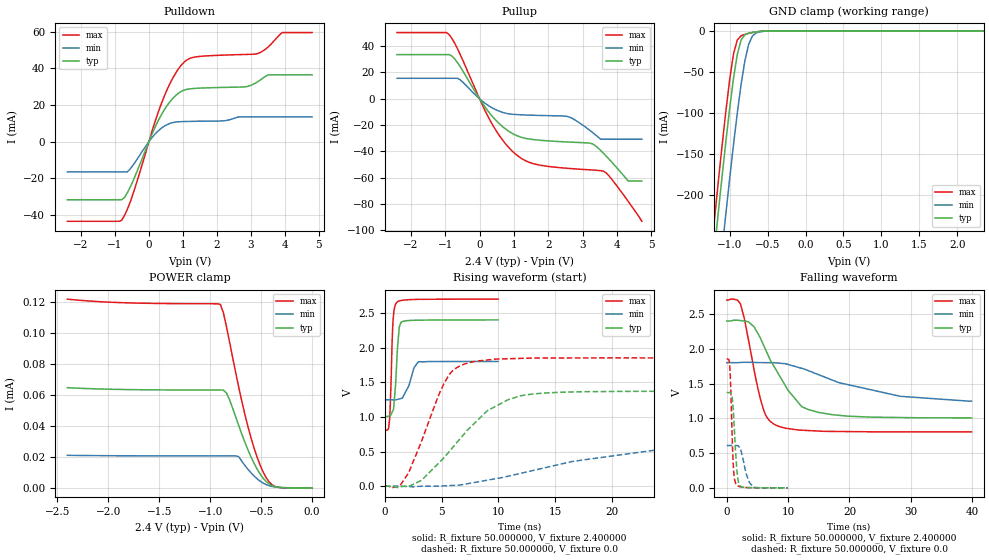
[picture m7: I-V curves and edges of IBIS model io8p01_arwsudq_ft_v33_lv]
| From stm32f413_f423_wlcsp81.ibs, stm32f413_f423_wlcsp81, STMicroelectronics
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|   Model io8p01_arwsudq_ft_v33_lv
[Model]  io8p01_arwsudq_ft_v33_lv
Model_type I/O
Polarity   Non-Inverting
Enable   Active-Low
Vinl =   0.720000V
Vinh =   1.680000V
Vmeas =  1.200000V
Cref =   50.000000pF
Rref =   100.000000M
Vref =   0.0V
C_comp   2.828400pF   2.771400pF   2.910300pF
[Temperature Range]   25.000000   0.125000k   -40.000000
[Pullup Reference]   2.400000V   1.800000V   2.700000V
[Pulldown Reference]   0.0V   0.0V   0.0V
[POWER Clamp Reference]   2.400000V   1.800000V   2.700000V
[GND Clamp Reference]   0.0V   0.0V   0.0V
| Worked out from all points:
|   slope of the pulldown table from 0 to 0.36 V, typ, clamps not added: 25 ohm
|   slope of the pullup table from 0 to 0.36 V, typ, clamps not added: 27.7 ohm
|   GND clamp passes 1 mA (typ) near -0.62 V on its own axis
|   rising waveform, R_fixture 50.000000, V_fixture 2.400000: 20-80 % time 323ps typ, 711ps min, 222ps max; typ from 1.01 V to 2.4 V
|   rising waveform, R_fixture 50.000000, V_fixture 0.0: 20-80 % time 4.72ns typ, 12.1ns min, 2.67ns max; typ from 0 V to 1.37 V
|   falling waveform, R_fixture 50.000000, V_fixture 2.400000: 20-80 % time 5.45ns typ, 13ns min, 2.68ns max; typ from 2.4 V to 1.01 V
|   falling waveform, R_fixture 50.000000, V_fixture 0.0: 20-80 % time 553ps typ, 1.05ns min, 408ps max; typ from 1.37 V to 0 V
[Pulldown]
|Voltage   I(typ)   I(min)   I(max)
-2.4V     -31.66mA   -16.51mA   -43.43mA
-800mV    -31.66mA   -16.51mA   -42.86mA
-480mV    -21.98mA   -13.17mA   -29.21mA
80mV      3.63mA     1.966mA    5.014mA
480mV     18.16mA    8.738mA    26.02mA
800mV     25.38mA    10.72mA    37.77mA
1.12V     28.53mA    11.02mA    44.6mA
2.8V      29.84mA    13.48mA    47.53mA
3.2V      32.65mA    13.48mA    48.04mA
3.52V     36.42mA    13.48mA    51.83mA
3.92V     36.42mA    13.48mA    59.49mA
4.8V      36.42mA    13.48mA    59.49mA
[Pullup]
|Voltage   I(typ)   I(min)   I(max)
-2.4V     33.57mA    15.57mA    50.34mA
-960mV    33.57mA    15.57mA    50.34mA
-800mV    32.45mA    15.57mA    45.78mA
-560mV    24.29mA    14.31mA    33.54mA
320mV     -11.75mA   -6.207mA   -17.08mA
960mV     -26.47mA   -11.82mA   -40.02mA
1.52V     -30.88mA   -12.51mA   -49.05mA
2.56V     -32.88mA   -13.49mA   -52.9mA
3.28V     -34.2mA    -25.51mA   -54.18mA
3.6V      -41.34mA   -30.76mA   -55mA
4.32V     -62.5mA    -30.76mA   -77.89mA
4.72V     -62.5mA    -30.76mA   -93.2mA
[GND_clamp]
|Voltage   I(typ)   I(min)   I(max)
-2.4V     -1.428A    -1.51A     -1.401A
-1.2V     -266.4mA   -356.3mA   -229.4mA
-1.15V    -221.3mA   -311mA     -184.1mA
-1.1V     -177.3mA   -266.4mA   -140mA
-1.05V    -134.8mA   -222.7mA   -97.97mA
-950mV    -58.22mA   -139.2mA   -28.55mA
-900mV    -29.03mA   -100.6mA   -11.27mA
-850mV    -11.41mA   -65.77mA   -6.067mA
-750mV    -2.852mA   -16.63mA   -3.179mA
-700mV    -1.914mA   -6.318mA   -2.181mA
-600mV    -750uA     -1.167mA   -738.3uA
2.35V     0A         0A         0A
[POWER_clamp]
|Voltage   I(typ)   I(min)   I(max)
-2.4V     64.71uA    21.03uA    121.9uA
-1.86V    63.55uA    20.74uA    119.6uA
-900mV    63.18uA    20.63uA    118.5uA
-870mV    63.14uA    20.63uA    113.2uA
-840mV    61.36uA    20.62uA    104.3uA
-720mV    40.37uA    20.18uA    65.28uA
-630mV    24.69uA    12.08uA    39.85uA
-540mV    12.26uA    5.907uA    20uA
-480mV    6.236uA    3.061uA    10.23uA
-420mV    2.4uA      1.365uA    3.726uA
-360mV    667.9nA    564nA      839.6nA
0V        0A         0A         0A
[Ramp]
| variable   typ   min   max
dV/dt_r  0.82218/4.71199n   0.38194/12.87085n   1.11102/2.66829n
dV/dt_f  0.83700/5.45997n   0.32238/13.04631n   1.13746/2.67925n
R_load = 50.000000
[Rising Waveform]
R_fixture= 50.000000
V_fixture= 2.400000
V_fixture_min= 1.800000
V_fixture_max= 2.700000
|time   V(typ)   V(min)   V(max)
0s        1.006V     1.247V     804.9mV
320.3ps   1.01V      1.247V     823.6mV
440.4ps   1.016V     1.247V     991.8mV
720.7ps   1.091V     1.247V     2.369V
940.9ps   1.445V     1.246V     2.621V
1.041ns   1.756V     1.249V     2.65V
1.281ns   2.299V     1.26V      2.673V
1.502ns   2.372V     1.269V     2.682V
2.963ns   2.396V     1.797V     2.697V
9.97ns    2.4V       1.8V       2.7V
[Rising Waveform]
R_fixture= 50.000000
V_fixture= 0.0
V_fixture_min= 0.0
V_fixture_max= 0.0
|time   V(typ)   V(min)   V(max)
0s        86.49uV    35.6uV     200.1uV
1.361ns   -9.084mV   -362.6uV   17.04mV
2.082ns   3.151mV    -5.824mV   188.3mV
3.283ns   91.99mV    -555.1uV   669.4mV
5.205ns   409.8mV    4.314mV    1.479V
7.047ns   764.9mV    28.95mV    1.765V
9.049ns   1.091V     87.12mV    1.822V
12.73ns   1.325V     214.6mV    1.848V
25.23ns   1.369V     552mV      1.851V
39.88ns   1.37V      609.1mV    1.851V
[Falling Waveform]
R_fixture= 50.000000
V_fixture= 2.400000
V_fixture_min= 1.800000
V_fixture_max= 2.700000
|time   V(typ)   V(min)   V(max)
0s        2.4V       1.8V       2.7V
2.242ns   2.405V     1.802V     2.643V
4.404ns   2.321V     1.804V     1.72V
5.526ns   2.146V     1.801V     1.264V
6.406ns   1.972V     1.8V       1.037V
7.768ns   1.737V     1.799V     912.8mV
12.17ns   1.171V     1.719V     829.1mV
14.89ns   1.086V     1.629V     817mV
28.27ns   1.011V     1.316V     805.2mV
39.88ns   1.006V     1.247V     804.9mV
[Falling Waveform]
R_fixture= 50.000000
V_fixture= 0.0
V_fixture_min= 0.0
V_fixture_max= 0.0
|time   V(typ)   V(min)   V(max)
0s        1.37V      609.1mV    1.851V
460.5ps   1.371V     609mV      1.791V
660.7ps   1.367V     608.9mV    1.414V
1.041ns   1.153V     608.6mV    369.2mV
1.481ns   469.9mV    609.7mV    59.58mV
1.822ns   121.3mV    606.3mV    27.36mV
2.282ns   20.78mV    550.6mV    14.27mV
3.143ns   4.871mV    207.7mV    5.64mV
4.364ns   2.142mV    9.617mV    1.752mV
9.97ns    86.49uV    35.6uV     200.1uV
